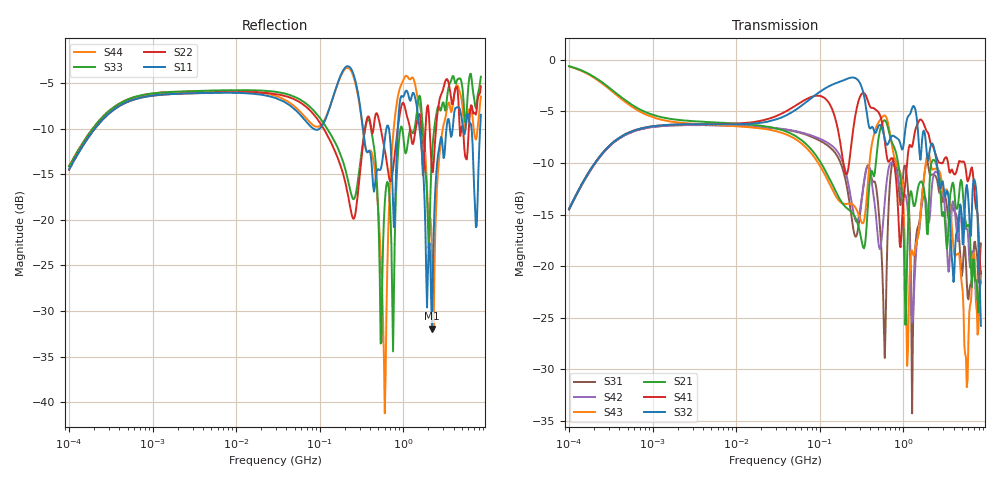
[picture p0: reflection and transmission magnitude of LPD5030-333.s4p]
# MHz S MA R 50
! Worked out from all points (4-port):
!   498 points, 100 kHz to 8.5 GHz, reference 50 ohm
!   strongest paths, dB at 100 kHz, 1.698 MHz, 29.49 MHz, 500.7 MHz, 8.5 GHz:
!     S32: -14.4, -6.3, -5.8, -6.5, -25.8
!     S41: -14.4, -6.3, -5.5, -5.0, -20.7
!     S21: -0.6, -5.7, -6.6, -7.8, -21.6
!     S43: -0.6, -6.0, -6.9, -6.1, -20.6
!     S42: -14.5, -6.3, -6.6, -17.5, -20.8
!     S31: -14.5, -6.4, -6.6, -14.0, -17.8
!   lowest |S11| = -31.9 dB at 2.209 GHz (marker M1), VSWR 1.05, Z = 49.7 - j2.5 ohm
!   |S11| at or under -10 dB: 329.1 MHz to 628.6 MHz (299.5 MHz wide, 62.5 % of centre); 1.567 GHz to 3.297 GHz (1.73 GHz wide, 71.1 % of centre); 6.566 GHz to 8.324 GHz (1.758 GHz wide, 23.6 % of centre)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
0.1  0.1891 65.3  0.9323 -10.8  0.1882 -113.5  0.1902 66.6
     0.9323 -10.8  0.1874 65.3  0.19 66.7  0.1887 -113.6
     0.1882 -113.5  0.19 66.7  0.1961 64.9  0.9288 -11.1
     0.1902 66.6  0.1887 -113.6  0.9288 -11.1  0.1974 65.4
220.0307  0.6938 -48.3  0.1885 119.4  0.2213 -4.7  0.2979 -20.9
          0.1885 119.4  0.1336 -62.3  0.8141 -38.6  0.2514 -4.5
          0.2213 -4.7  0.8141 -38.6  0.1612 -62.5  0.2011 106.8
          0.2979 -20.9  0.2514 -4.5  0.2011 106.8  0.6791 -55.4
601.0223  0.2744 -77.8  0.5099 -47.0  0.03595 142.5  0.4057 -121.2
          0.5099 -47.0  0.2415 -165.6  0.4141 -104.8  0.206 -38.5
          0.03595 142.5  0.4141 -104.8  0.1236 -47.6  0.5378 -65.5
          0.4057 -121.2  0.206 -38.5  0.5378 -65.5  0.00869 147.2
1016.278  0.4765 -143.8  0.1328 138.3  0.297 -121.5  0.2183 -109.6
          0.1328 138.3  0.4321 -100.1  0.3973 -135.2  0.219 -163.7
          0.297 -121.5  0.3973 -135.2  0.2677 -109.3  0.1785 139.0
          0.2183 -109.6  0.219 -163.7  0.1785 139.0  0.5915 -119.9
2209.207  0.02527 -96.4  0.3219 95.6  0.2784 76.0  0.3877 54.8
          0.3219 95.6  0.1849 85.0  0.3947 36.5  0.2457 102.3
          0.2784 76.0  0.3947 36.5  0.226 142.6  0.2951 78.7
          0.3877 54.8  0.2457 102.3  0.2951 78.7  0.06377 -1.1
6920.76  0.1921 -175.2  0.1085 -172.8  0.1121 -149.7  0.2659 141.4
         0.1085 -172.8  0.3814 -158.1  0.2605 163.7  0.1177 162.3
         0.1121 -149.7  0.2605 163.7  0.487 -175.2  0.1143 -127.6
         0.2659 141.4  0.1177 162.3  0.1143 -127.6  0.3247 -166.3
8500  0.3761 -16.6  0.08332 -2.9  0.1291 13.2  0.09239 -70.2
      0.08332 -2.9  0.538 -24.0  0.05145 -153.2  0.09156 12.4
      0.1291 13.2  0.05145 -153.2  0.6082 -34.1  0.0936 38.1
      0.09239 -70.2  0.09156 12.4  0.0936 38.1  0.4732 -28.1
